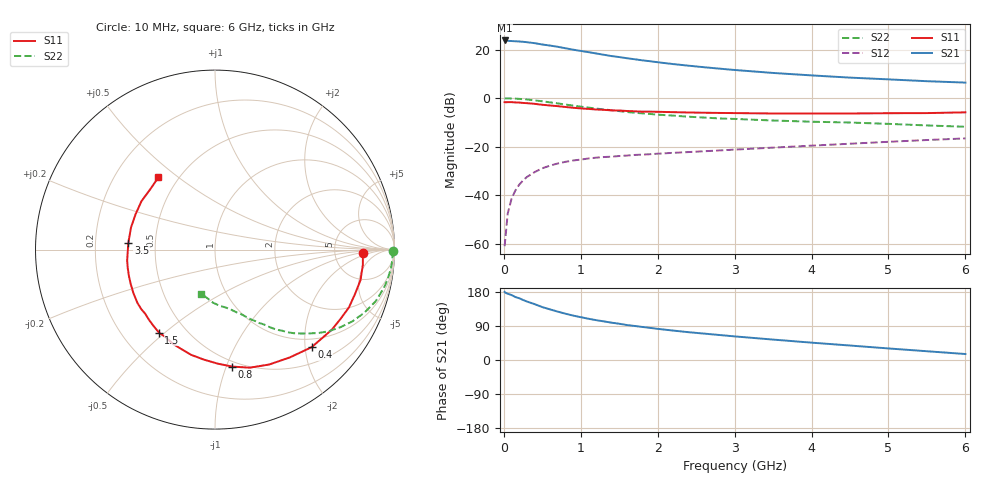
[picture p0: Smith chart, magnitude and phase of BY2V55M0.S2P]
! SIEMENS Small Signal Semiconductors
! BFY420
! Si NPN RF SIEGET Grounded Emitter Transistor in MICRO-X
! VCE = 2.5 V  IC = 5 mA
! Common Emitter S-Parameters:  October  1996
# GHz  S  MA  R  50
!  f  S11  S21  S12  S22
! GHz  MAG  ANG  MAG  ANG  MAG  ANG  MAG  ANG
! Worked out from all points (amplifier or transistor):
!   36 points, 10 MHz to 6 GHz, reference 50 ohm
!   highest |S21| = 23.8 dB at 10 MHz (marker M1)
!   |S21| within 3 dB of that: start of sweep to 766.1 MHz
!   unconditionally stable (mu >= 1): 3.17 GHz to end of sweep
!   at 250 MHz: K = 0.11, MSG = 28.5 dB, |S12| = -33.9 dB
!   at 1.4 GHz: K = 0.53, MSG = 20.7 dB, |S12| = -24.1 dB
!   at 6 GHz: K = 1.14, MAG = 9.2 dB, |S12| = -16.6 dB
!   S11 on the Smith chart (normalised r, x): 10 MHz: 10, -1; 400 MHz: 0.81, -2.14; 800 MHz: 0.46, -1.05; 1.5 GHz: 0.36, -0.48; 3.5 GHz: 0.35, +0.03; 6 GHz: 0.39, +0.43
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0.01  0.8276 -1.4  15.42 179.9  0.0009 94.0  0.9919 -0.5
0.02  0.8246 -2.5  15.38 177.6  0.0013 86.0  0.9883 -1.2
0.05  0.8281 -5.9  15.1 174.9  0.0042 88.3  0.9903 -3.0
0.1  0.8284 -11.8  15.01 171.5  0.0085 84.6  0.9856 -6.2
0.15  0.8184 -17.6  14.83 166.2  0.0126 80.3  0.977 -9.2
0.2  0.8127 -23.4  14.68 162.9  0.0166 77.9  0.9678 -12.0
0.3  0.7889 -34.5  14.2 154.3  0.0239 72.6  0.9405 -17.8
0.4  0.7652 -45.3  13.56 147.4  0.0301 67.0  0.9028 -23.0
0.5  0.731 -55.3  12.73 139.6  0.0361 62.0  0.8625 -27.7
0.6  0.7079 -64.7  12.1 133.6  0.0409 58.6  0.8212 -31.8
0.8  0.6589 -81.6  10.66 122.2  0.049 51.5  0.7402 -38.9
0.9  0.6357 -88.6  9.967 117.2  0.0522 49.1  0.7031 -41.6
1.1  0.6014 -102.7  8.868 108.9  0.0574 45.2  0.6401 -46.7
1.3  0.5757 -113.7  7.825 101.9  0.0615 42.2  0.586 -50.4
1.5  0.5578 -124.1  7.022 95.7  0.0645 40.1  0.5414 -53.9
1.8  0.5281 -137.4  6.009 87.2  0.0689 38.6  0.4872 -57.9
2.2  0.5156 -151.7  5.036 77.7  0.075 36.7  0.4377 -62.7
2.8  0.4969 -168.0  4.059 66.0  0.084 35.2  0.3829 -68.7
3.5  0.4844 175.6  3.306 53.9  0.096 33.8  0.3471 -74.9
4.5  0.4844 156.0  2.65 38.2  0.1155 30.0  0.3152 -84.9
5.5  0.4931 137.0  2.236 23.1  0.1377 24.7  0.2747 -98.7
6  0.5113 128.1  2.093 15.8  0.1486 21.5  0.258 -107.2
